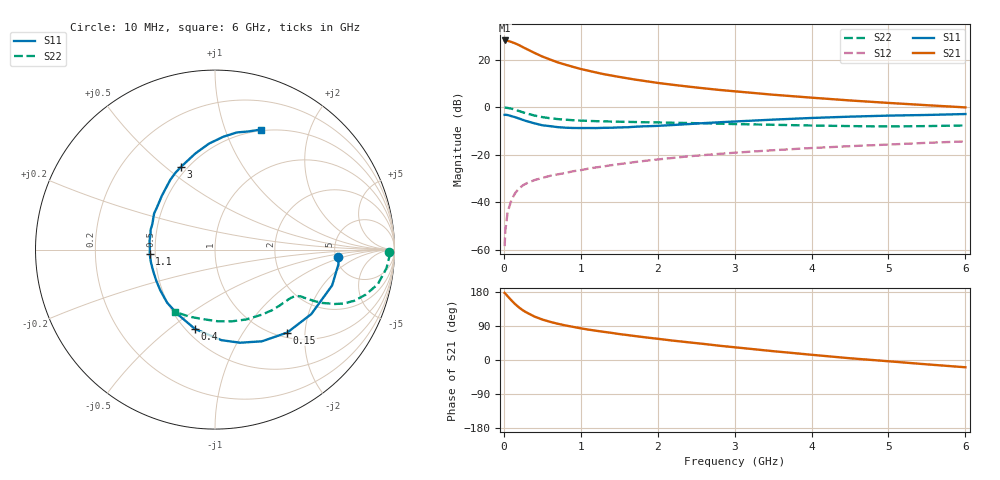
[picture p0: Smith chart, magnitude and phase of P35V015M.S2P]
! SIEMENS Small Signal Semiconductors
! BFP181
! Si NPN RF Bipolar Junction Transistor in SOT143
! VCE = 5 V  IC = 15 mA
! Common Emitter S-Parameters:  March  1996
# GHz  S  MA  R  50
!  f  S11  S21  S12  S22
! GHz  MAG  ANG  MAG  ANG  MAG  ANG  MAG  ANG
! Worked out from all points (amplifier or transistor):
!   36 points, 10 MHz to 6 GHz, reference 50 ohm
!   highest |S21| = 28.0 dB at 10 MHz (marker M1)
!   |S21| within 3 dB of that: start of sweep to 259 MHz
!   unconditionally stable (mu >= 1): 945.6 MHz to 5.987 GHz
!   at 250 MHz: K = 0.41, MSG = 29.0 dB, |S12| = -32.8 dB
!   at 1.4 GHz: K = 1.13, MAG = 16.7 dB, |S12| = -24.4 dB
!   at 6 GHz: K = 1.00, MSG = 7.1 dB, |S12| = -14.4 dB
!   S11 on the Smith chart (normalised r, x): 10 MHz: 5.29, -0.85; 150 MHz: 1.09, -1.62; 400 MHz: 0.55, -0.62; 1.1 GHz: 0.47, -0.03; 3 GHz: 0.46, +0.57; 6 GHz: 0.49, +1.34
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0.01  0.6892 -3.5  25.16 177.0  0.0012 85.0  0.9704 -0.9
0.02  0.6924 -6.8  25.07 175.2  0.0026 85.8  0.9723 -2.3
0.05  0.6824 -17.0  24.72 168.0  0.0063 85.0  0.9611 -6.2
0.1  0.6457 -33.8  23.34 157.1  0.0114 74.0  0.9273 -12.0
0.15  0.6128 -49.0  21.76 146.9  0.0159 68.0  0.877 -16.6
0.2  0.574 -62.9  19.99 138.2  0.0197 63.6  0.8263 -20.2
0.25  0.5374 -74.9  18.11 130.8  0.0229 60.2  0.776 -22.8
0.3  0.506 -85.9  16.51 124.9  0.0253 57.4  0.7334 -24.4
0.4  0.4562 -104.1  13.75 114.5  0.0294 54.5  0.6654 -26.5
0.5  0.4161 -119.8  11.57 106.8  0.0326 52.3  0.6175 -27.5
0.6  0.3984 -132.0  10.03 100.8  0.036 52.0  0.5846 -28.0
0.7  0.3798 -143.5  8.72 95.7  0.0387 52.5  0.5614 -28.4
0.9  0.3648 -160.5  7.013 87.4  0.045 52.8  0.5313 -29.2
1.1  0.3644 -175.9  5.813 80.2  0.0511 53.1  0.5137 -30.5
1.3  0.368 172.6  4.927 74.3  0.0569 52.8  0.5023 -32.3
1.6  0.3772 157.5  4.05 66.0  0.0666 52.3  0.4905 -35.4
2.2  0.421 134.8  2.943 51.1  0.0858 49.7  0.4698 -43.6
3  0.499 112.2  2.151 33.6  0.1102 44.1  0.441 -56.6
3.5  0.5464 101.6  1.823 23.3  0.1244 40.5  0.426 -66.1
4.5  0.6309 85.7  1.381 4.6  0.1513 32.5  0.3996 -87.9
5.5  0.6847 74.1  1.098 -11.5  0.1779 25.1  0.3999 -110.8
6  0.7165 69.0  0.987 -19.2  0.1908 20.9  0.4124 -122.6
